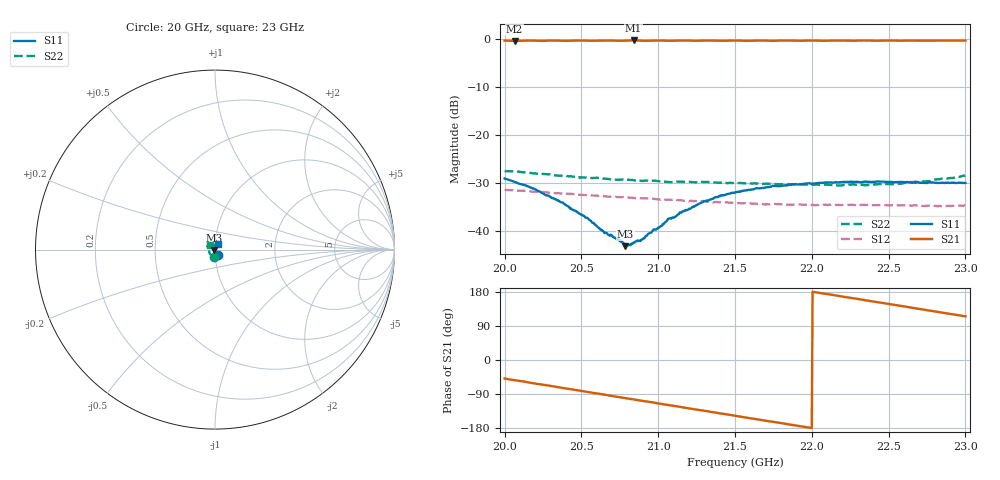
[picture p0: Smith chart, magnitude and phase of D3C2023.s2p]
! 11/6/2020 9:52:02 AM
! C:\USERS\DITOM\DESKTOP\SINGLE JUNCTION ISOLATOR DATA\20.0 - 23.0 GHZ (D3I2023).S2P
! CHANNEL.1
! TR.MEASUREMENT
! CORRECTED.DATA
# GHZ S RI R 50.0
! FREQ.GHZ  S11RE  S11IM  S21RE  S21IM  S12RE  S12IM  S22RE  S22IM
!; PortSelection: Port_12
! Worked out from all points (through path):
!   601 points, 20 GHz to 23 GHz, reference 50 ohm
!   highest |S21| = -0.21 dB at 20.84 GHz (marker M1); lowest = -0.3 dB at 20.07 GHz (marker M2)
!   lowest |S11| = -43.1 dB at 20.79 GHz (marker M3), VSWR 1.01, Z = 49.3 - j0.176 ohm
!   |S11| at or under -10 dB: start of sweep to end of sweep
!   |S22| runs from -30.5 to -27.4 dB; largest |S21 - S12| = 0.99
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20  0.0158 -0.0318  0.6405 -0.7329  -0.027 -0.00333  -0.00656 -0.0421
20.065  0.013 -0.0302  0.5769 -0.7733  -0.0267 -0.00158  -0.0099 -0.0409
20.19  0.00806 -0.0266  0.4608 -0.8544  -0.0259 0.00117  -0.0153 -0.0371
20.32  0.00319 -0.0219  0.3346 -0.9151  -0.0247 0.004  -0.0203 -0.0327
20.5  -0.00232 -0.0147  0.1385 -0.9642  -0.023 0.00739  -0.0262 -0.0253
20.64  -0.00521 -0.00873  -0.0138 -0.9723  -0.0213 0.00977  -0.0297 -0.0197
20.785  -0.00678 -0.00179  -0.1709 -0.9551  -0.0193 0.0117  -0.0322 -0.0127
20.805  -0.00698 -0.00151  -0.1939 -0.9534  -0.0191 0.012  -0.0324 -0.012
20.84  -0.00759 0.000313  -0.2375 -0.9469  -0.0186 0.0124  -0.0325 -0.0103
20.895  -0.00778 0.00266  -0.2962 -0.9219  -0.0179 0.0131  -0.0329 -0.00775
21  -0.00798 0.00747  -0.404 -0.8876  -0.0162 0.0142  -0.0333 -0.0034
21.075  -0.00774 0.0112  -0.4755 -0.8438  -0.0152 0.015  -0.0326 -0.000163
21.285  -0.00468 0.0195  -0.6616 -0.711  -0.0118 0.017  -0.0317 0.00816
21.5  0.000603 0.0254  -0.817 -0.5299  -0.00821 0.018  -0.0286 0.0141
21.69  0.00533 0.028  -0.9123 -0.3392  -0.00524 0.0184  -0.0258 0.0178
21.835  0.00827 0.0292  -0.9562 -0.1871  -0.00269 0.0188  -0.0238 0.02
22  0.011 0.0292  -0.974 -0.00629  -7.89e-05 0.0189  -0.0219 0.0212
22.17  0.0134 0.0295  -0.9568 0.1796  0.00313 0.0186  -0.0205 0.0221
22.305  0.0143 0.0293  -0.9186 0.3203  0.00558 0.018  -0.0207 0.0227
22.5  0.0155 0.029  -0.8251 0.5187  0.0093 0.0162  -0.0211 0.0229
22.715  0.0152 0.0283  -0.6718 0.7027  0.0128 0.0132  -0.0228 0.0234
23  0.0143 0.0287  -0.4145 0.8802  0.0167 0.00813  -0.0277 0.0263
